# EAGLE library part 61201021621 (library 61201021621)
10 way 2.54mm male box Header Wurth Elektronik 612 Series, 2.54mm Pitch 10 Way 2 Row Straight PCB Header, Solder Termination, 3A Source: Datasheet
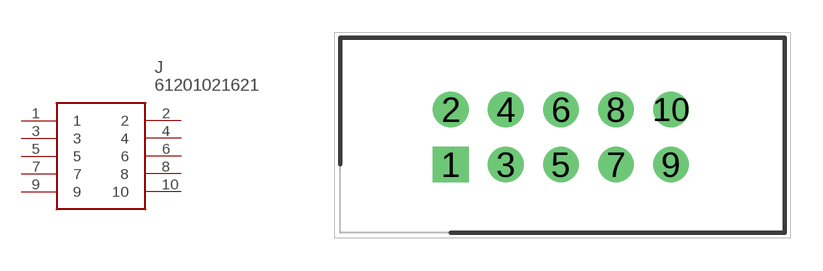
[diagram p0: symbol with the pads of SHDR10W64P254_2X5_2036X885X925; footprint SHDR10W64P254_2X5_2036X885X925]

Designator prefix J

## 61201021621 (Description: 10 way 2.54mm male box Header Wurth Elektronik 612 Series, 2.54mm Pitch 10 Way 2 Row Straight PCB Header, Solder Termination, 3A; Height: 9.25mm; Manufacturer_Name: Wurth Elektronik; Manufacturer_Part_Number: 61201021621; Mouser_Part_Number: 710-61201021621; Mouser_Price-Stock: https://www.mouser.co.uk/ProductDetail/Wurth-Elektronik/61201021621?qs=W%252B2sBeLta1a0dwX5pxbfXw%3D%3D)  [SHDR10W64P254_2X5_2036X885X925]
1  1
2  2
3  3
4  4
5  5
6  6
7  7
8  8
9  9
10  10

## Footprint SHDR10W64P254_2X5_2036X885X925 (pad centres in mm)
61201021621
drill 1.1 pad 1.65 square: 1 0,0
drill 1.1 pad 1.65: 2 0,2.54; 3 2.54,0; 4 2.54,2.54; 5 5.08,0; 6 5.08,2.54; 7 7.62,0; 8 7.62,2.54; 9 10.16,0; 10 10.16,2.54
